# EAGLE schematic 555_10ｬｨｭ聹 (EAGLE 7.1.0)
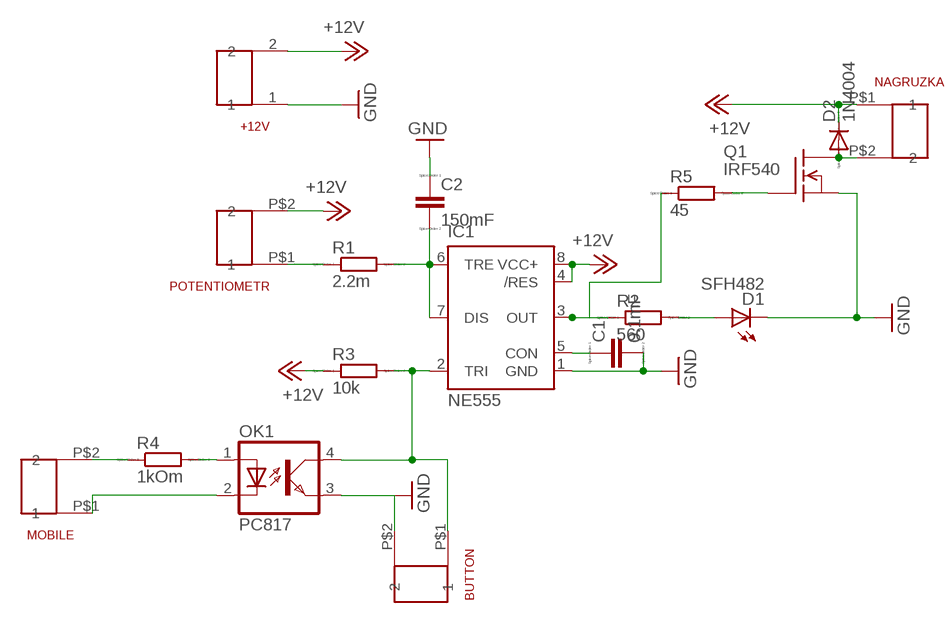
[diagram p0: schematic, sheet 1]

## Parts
+12V  CON2X2.54  [CON2X2.54]
BUTTON  CON2X3.4  [CON2X3.4]
C1  0.1mF  C-EU025-024X044  [C025-024X044]
C2  150mF  C-EU025-024X044  [C025-024X044]
D1  SFH482  [SFH482]
D2  1N4004  [DO41-10]
IC1  NE555  [DIL-08]
MOBILE  CON2X3.4  [CON2X3.4]
NAGRUZKA  CON2X3.4  [CON2X3.4]
OK1  PC817  [DIL04]
POTENTIOMETR  CON2X3.4  [CON2X3.4]
Q1  IRF540  [TO220]
R1  2.2m  R-EU_0204_2V  [0204V]
R2  560  R-EU_0204_2V  [0204V]
R3  10k  R-EU_0204_2V  [0204V]
R4  1kOm  R-EU_0204_2V  [0204V]
R5  45  R-EU_0204_2V  [0204V]

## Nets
+12V: +12V.2 D2.C IC1.4(/RES) IC1.8(VCC+) NAGRUZKA.P$1 POTENTIOMETR.P$2 R3.1
GND: +12V.1 BUTTON.P$2 C1.2 C2.1 D1.K(C) IC1.1(GND) OK1.3(EMIT) Q1.3(S)
N$1: C2.2 IC1.6(TRE) IC1.7(DIS) R1.2
N$2: POTENTIOMETR.P$1 R1.1
N$3: MOBILE.P$2 R4.1
N$4: IC1.3(OUT) R2.1 R5.1
N$5: D1.A R2.2
N$6: BUTTON.P$1 IC1.2(TRI) OK1.4(COL) R3.2
N$7: C1.1 IC1.5(CON)
N$8: OK1.1(A) R4.2
N$9: MOBILE.P$1 OK1.2(C)
N$11: Q1.1(G) R5.2
N$12: D2.A NAGRUZKA.P$2 Q1.2(D)

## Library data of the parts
+12V = my:CON2X2.54
BUTTON MOBILE NAGRUZKA POTENTIOMETR = my:CON2X3.4
C1 C2 = resistor:C-EU: CAPACITOR, European symbol; SPICEPREFIX: C
D1 = led:SFH482: IR LED
D2 = diode:1N4004: DIODE
IC1 = st-microelectronics:NE555: General purpose bipolar Timer; MF: Arrow Electronics; MPN: NE555N; OC_FARNELL: 1467742; OC_NEWARK: 89K1486
OK1 = optocoupler:PC817: SHARP OPTO COUPLER; MPN: PC817X4J000F; OC_FARNELL: 9707727; OC_NEWARK: 97K7059
Q1 = transistor-fet:IRF540: N-Channel Enhancement MOSFET (HEXFET); 100V; 28A; 0,077Ohm
R1-R5 = resistor:R-EU_: RESISTOR, European symbol; SPICEPREFIX: R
